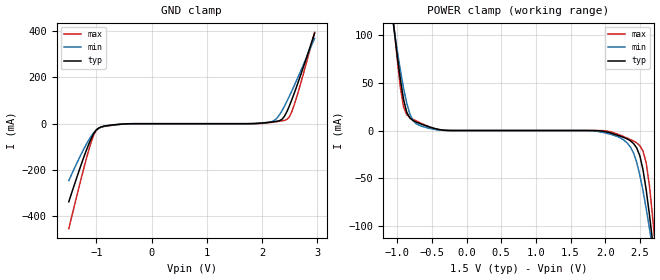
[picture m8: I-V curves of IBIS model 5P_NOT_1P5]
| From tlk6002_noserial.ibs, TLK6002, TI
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[Model]   5P_NOT_1P5
Model_type   Input
Polarity   Non-Inverting
Vinh =  0.85
Vinl =  0.65
C_comp   2.108887p   1.924381p   2.428843p
[Model Spec]
Vinh   0.85   0.8125   0.8875
Vinl   0.65   0.6125   0.6875
[Temperature Range]   25   125   -40
[Voltage Range]   1.5   1.425   1.575
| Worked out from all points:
|   GND clamp passes 1 mA (typ) near -0.48 V on its own axis
|   POWER clamp passes 1 mA (typ) near -0.39 V on its own axis
[POWER_clamp]
-1.5V     423.5mA    352.2mA    503mA
-1.045V   105.8mA    105.4mA    107.7mA
-909.1mV  32.54mA    44.27mA    24.77mA
-772.7mV  10.47mA    10.51mA    11.79mA
-590.9mV  5.058mA    3.284mA    5.458mA
1.909V    -271uA     -1.151mA   -27.39uA
2.273V    -7.41mA    -10.27mA   -6.593mA
2.455V    -18.25mA   -33.42mA   -12.88mA
2.591V    -62.1mA    -81.63mA   -33.73mA
2.682V    -114.8mA   -122.6mA   -88.81mA
2.727V    -144.2mA   -144.5mA   -125.6mA
2.955V    -303.7mA   -261.3mA   -335.5mA
[GND_clamp]
-1.5V     -337mA     -245.7mA   -453.6mA
-1.136V   -87.16mA   -69.43mA   -112.3mA
-1.045V   -41.26mA   -37.73mA   -47.59mA
-954.5mV  -18.25mA   -19.11mA   -19.1mA
-409.1mV  -271uA     -435uA     -205.3uA
2.136V    6.262mA    6.46mA     4.557mA
2.273V    10.47mA    24.1mA     9.048mA
2.364V    19.13mA    56.1mA     12.41mA
2.455V    53.09mA    97.61mA    18.35mA
2.5V      78.14mA    120.2mA    30.37mA
2.591V    135.1mA    167.4mA    85.29mA
2.955V    390.4mA    369mA      394.5mA
